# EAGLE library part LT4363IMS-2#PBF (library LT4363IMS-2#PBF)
High Voltage Surge Stopper with Current Limit Source: Datasheet
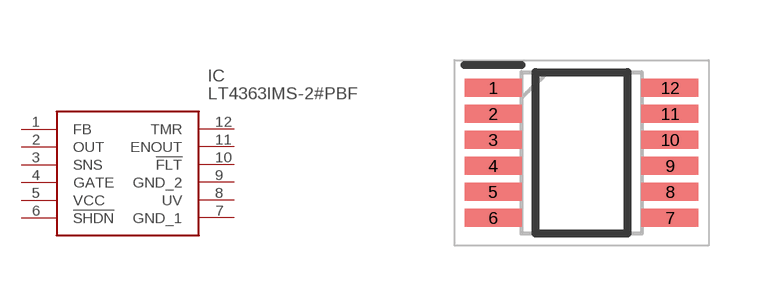
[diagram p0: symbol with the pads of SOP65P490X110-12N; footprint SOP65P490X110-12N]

Designator prefix IC

## LT4363IMS-2#PBF (Description: High Voltage Surge Stopper with Current Limit; Height: 1.1mm; Manufacturer_Name: Analog Devices; Manufacturer_Part_Number: LT4363IMS-2#PBF; Mouser_Part_Number: 584-LT4363IMS-2#PBF; Mouser_Price-Stock: https://www.mouser.co.uk/ProductDetail/Analog-Devices/LT4363IMS-2PBF?qs=hVkxg5c3xu8ajQHTH9qgCg%3D%3D)  [SOP65P490X110-12N]
1  FB
2  OUT
3  SNS
4  GATE
5  VCC
6  !SHDN
7  GND_1
8  UV
9  GND_2
10  !FLT
11  ENOUT
12  TMR

## Footprint SOP65P490X110-12N (pad centres in mm)
12-Lead Plastic MSOP
smd 1.425 x 0.45: 1 -2.212,1.625; 2 -2.212,0.975; 3 -2.212,0.325; 4 -2.212,-0.325; 5 -2.212,-0.975; 6 -2.212,-1.625; 7 2.212,-1.625; 8 2.212,-0.975; 9 2.212,-0.325; 10 2.212,0.325; 11 2.212,0.975; 12 2.212,1.625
